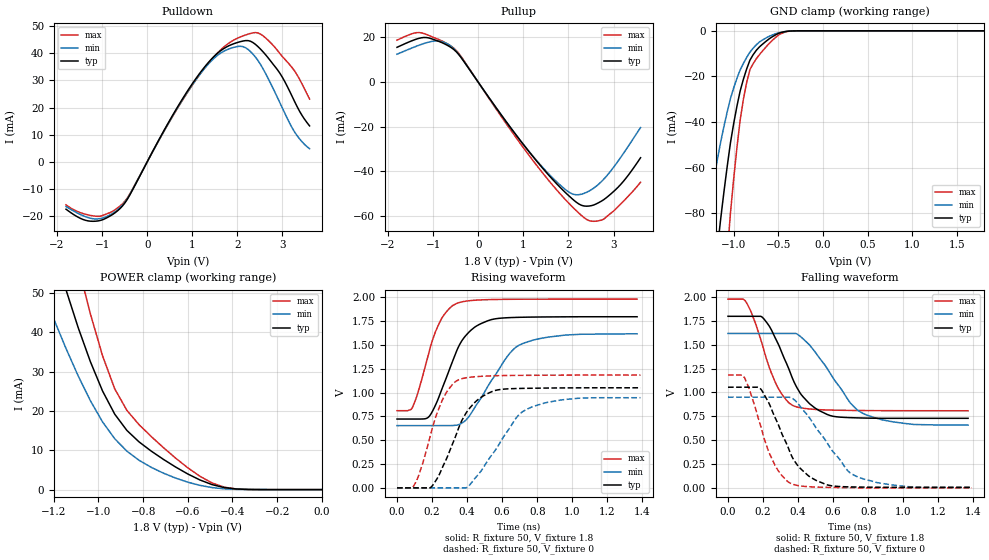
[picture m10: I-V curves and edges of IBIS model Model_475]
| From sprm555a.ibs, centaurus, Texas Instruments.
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| Model based on original model for BCSHTLTCSCDDVPBFZ_SSGFV
|   Sub model SR01_11MA_PADN_10PER_1P8
[model]   Model_475
|[Description]  [1.8V-3-STATE-X-FAST:11MA, IND, 10%]
|   Fast slew rate (SR[1:0] = "10"), 0.73 * RExt = 1.325 * Iout
|   (I[2:0] = "110"), 11mA nominal with Rext = 50R, ,Industrial
|   temperature range (-40C to 125C, 25C nominal),10% power supply
|   tolerance
|[Input Load]
|[Output Drive] FAST:11MA
|Voltage   1.8V
|Mode   3-STATE
Model_type   3-state
Polarity   Non-Inverting
Enable   Active-Low
Cref =  15pF
Rref =  100.0000M
Vref =  0V
Vmeas =  0.9
C_comp   1.851324p   1.663768p   1.973575p
[Temperature Range]   25   125   -40
[Voltage Range]   1.8   1.62   1.98
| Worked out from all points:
|   slope of the pulldown table from 0 to 0.27 V, typ, clamps not added: 32 ohm
|   slope of the pullup table from 0 to 0.27 V, typ, clamps not added: 34.5 ohm
|   GND clamp passes 1 mA (typ) near -0.49 V on its own axis
|   POWER clamp passes 1 mA (typ) near -0.47 V on its own axis
|   rising waveform, R_fixture 50, V_fixture 1.8: 20-80 % time 149ps typ, 205ps min, 120ps max; typ from 0.722 V to 1.79 V
|   rising waveform, R_fixture 50, V_fixture 0: 20-80 % time 158ps typ, 206ps min, 123ps max; typ from 0 V to 1.05 V
|   falling waveform, R_fixture 50, V_fixture 1.8: 20-80 % time 168ps typ, 223ps min, 135ps max; typ from 1.8 V to 0.729 V
|   falling waveform, R_fixture 50, V_fixture 0: 20-80 % time 163ps typ, 223ps min, 131ps max; typ from 1.05 V to 0.004 V
[POWER_clamp]
-1.8V     194.9mA    137.1mA    262.8mA
-1.236V   68.49mA    48.51mA    92.67mA
-1.145V   50.76mA    35.86mA    69.65mA
-1.127V   47.56mA    33.54mA    65.34mA
-1.055V   35.4mA     24.69mA    48.69mA
-981.8mV  25.06mA    17.2mA     34.01mA
-927.3mV  19.17mA    12.93mA    25.61mA
-872.7mV  15.03mA    9.767mA    20.12mA
-818.2mV  12.12mA    7.45mA     16.5mA
-654.5mV  5.738mA    2.93mA     8.003mA
-436.4mV  508.2uA    199.4uA    613uA
0V        2.273nA    15.95nA    16.67nA
[Pulldown]
-1.8V     -17.41mA   -16.43mA   -15.81mA
-1.145V   -21.83mA   -21.01mA   -19.99mA
-545.5mV  -16.18mA   -15.87mA   -15.39mA
545.5mV   16.61mA    16.34mA    16.22mA
1.091V    30.91mA    30.47mA    30.41mA
1.527V    39.51mA    38.78mA    39.54mA
1.964V    43.74mA    42.34mA    45.21mA
2.291V    44.39mA    40.59mA    47.27mA
2.618V    39.56mA    32.74mA    45.71mA
2.945V    32.54mA    21.66mA    39.78mA
3.218V    23.95mA    12.39mA    34.58mA
3.6V      13.24mA    4.837mA    23.12mA
[Pullup]
-1.8V     15.59mA    12.51mA    18.8mA
-1.309V   19.63mA    16.55mA    22.2mA
-927.3mV  18.65mA    18.46mA    19.52mA
-600mV    15.48mA    16.08mA    16.11mA
-381.8mV  11.09mA    11.19mA    11.57mA
1.2V      -32.98mA   -32.79mA   -34.72mA
1.745V    -45.62mA   -44.74mA   -48.37mA
2.127V    -52.98mA   -50.3mA    -56.63mA
2.455V    -55.48mA   -48.79mA   -61.96mA
2.727V    -53.34mA   -44.61mA   -61.81mA
3.164V    -45.71mA   -33.58mA   -54.45mA
3.6V      -33.84mA   -20.34mA   -44.81mA
[GND_clamp]
-1.8V     -346.1mA   -209.3mA   -568.3mA
-1.327V   -149.7mA   -89.03mA   -250.9mA
-1.291V   -135.6mA   -80.47mA   -227.5mA
-1.145V   -82.35mA   -48.67mA   -137.7mA
-1.073V   -59.44mA   -35.55mA   -97.96mA
-1.036V   -49.1mA    -29.72mA   -79.9mA
-927.3mV  -26.31mA   -17.11mA   -38.99mA
-854.5mV  -16.67mA   -11.64mA   -22.56mA
-818.2mV  -12.86mA   -9.351mA   -16.98mA
-672.7mV  -5.705mA   -3.913mA   -8.624mA
-381.8mV  -120.4uA   -129uA     -167.4uA
1.8V      2.273nA    454nA      6.646nA
[Ramp]
dV/dt_f 0.64847465/0.17112877n 0.58181524/0.22275036n 0.70398464/0.1348948n
dV/dt_r 0.63533858/0.15998065n 0.57312974/0.20794216n 0.71186492/0.12296955n
R_load = 50
[Rising Waveform]
R_fixture = 50
V_fixture = 1.8
V_fixture_min = 1.62
V_fixture_max = 1.98
0s        722mV      653mV      809.4mV
88.2ps    722mV      653mV      845mV
184.9ps   752.4mV    653mV      1.439V
256.8ps   1.039V     653.2mV    1.783V
341ps     1.44V      657.8mV    1.935V
395.8ps   1.605V     715.3mV    1.959V
468.3ps   1.713V     911.4mV    1.971V
693.4ps   1.789V     1.494V     1.979V
959.3ps   1.794V     1.603V     1.98V
1.37ns    1.795V     1.616V     1.98V
[Rising Waveform]
R_fixture = 50
V_fixture = 0
V_fixture_min = 0
V_fixture_max = 0
0s        0V         0V         0V
93.9ps    0V         0V         16.56mV
198.8ps   15.99mV    0V         608.1mV
268.7ps   252mV      0V         957.4mV
350ps     619.3mV    0V         1.132V
404.3ps   812.2mV    11.48mV    1.158V
492.7ps   964.8mV    211.9mV    1.171V
677.8ps   1.042V     727.9mV    1.18V
743.6ps   1.044V     827mV      1.181V
1.39ns    1.05V      945.6mV    1.184V
[Falling Waveform]
R_fixture = 50
V_fixture = 1.8
V_fixture_min = 1.62
V_fixture_max = 1.98
0s        1.799V     1.619V     1.979V
98.6ps    1.799V     1.619V     1.961V
197ps     1.787V     1.619V     1.494V
278.3ps   1.539V     1.619V     1.073V
369.5ps   1.141V     1.619V     864mV
419.5ps   974mV      1.578V     837.7mV
522ps     808.4mV    1.361V     819.8mV
765.9ps   732.5mV    783.9mV    810.7mV
1.06ns    729.3mV    664.5mV    808.8mV
1.37ns    729.3mV    658.5mV    808.5mV
[Falling Waveform]
R_fixture = 50
V_fixture = 0
V_fixture_min = 0
V_fixture_max = 0
0s        1.055V     951.4mV    1.183V
94.3ps    1.055V     951.4mV    1.155V
188.2ps   1.034V     951.4mV    638.1mV
268.1ps   738.1mV    951.4mV    236.6mV
361.1ps   342.2mV    944mV      44.18mV
404.3ps   218.9mV    871.5mV    22.9mV
504.3ps   76.78mV    624.7mV    8.302mV
716.2ps   9.26mV     135.3mV    2.139mV
1.018ns   5.126mV    13.23mV    0V
1.39ns    4.188mV    6.954mV    0V
